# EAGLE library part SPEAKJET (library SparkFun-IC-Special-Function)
Speech synthesis chip User Manual SparkFun Products SpeakJet (COM-09578)
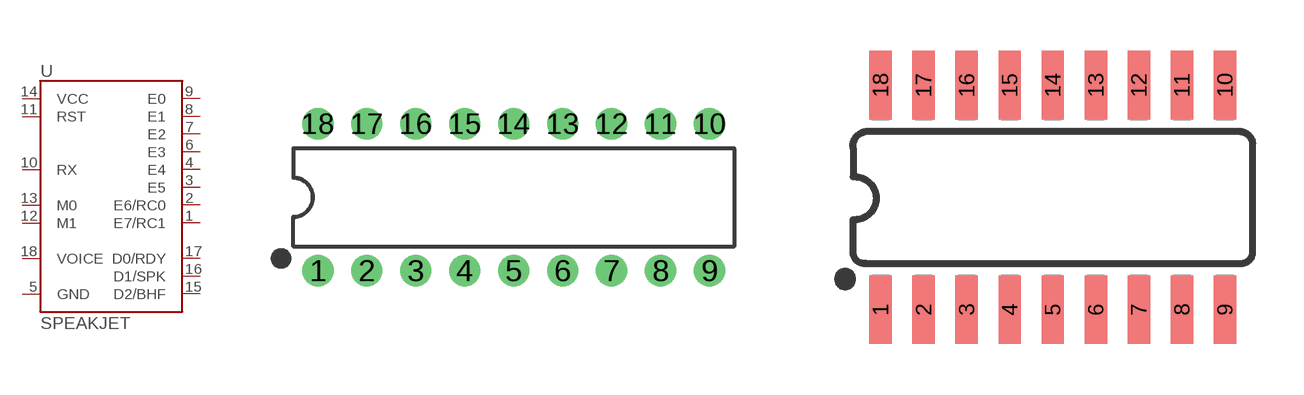
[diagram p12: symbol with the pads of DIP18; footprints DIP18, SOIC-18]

Designator prefix U

## SPEAKJETDIP (PROD_ID: IC-09512; VALUE: SPEAKJET)  [DIP18]
1  E7/RC1
2  E6/RC0
3  E5
4  E4
5  GND
6  E3
7  E2
8  E1
9  E0
10  RX
11  RST
12  M1
13  M0
14  VCC
15  D2/BHF
16  D1/SPK
17  D0/RDY
18  VOICE

## SPEAKJETSMD (PROD_ID: IC-XXXXX; VALUE: SPEAKJET)  [SOIC-18]
Pads as for DIP18

## Footprint DIP18 (pad centres in mm)
Dual In Line package type P
drill 0.813 pad 1.626: 1 -10.16,-3.81; 2 -7.62,-3.81; 3 -5.08,-3.81; 4 -2.54,-3.81; 5 0,-3.81; 6 2.54,-3.81; 7 5.08,-3.81; 8 7.62,-3.81; 9 10.16,-3.81; 10 10.16,3.81; 11 7.62,3.81; 12 5.08,3.81; 13 2.54,3.81; 14 0,3.81; 15 -2.54,3.81; 16 -5.08,3.81; 17 -7.62,3.81; 18 -10.16,3.81

## Footprint SOIC-18 (pad centres in mm)
smd 0.66 x 2.032: 1 -7.685,-3.285; 2 -6.415,-3.285; 3 -5.145,-3.285; 4 -3.875,-3.285; 5 -2.605,-3.285; 6 -1.335,-3.285; 7 -0.065,-3.285; 8 1.205,-3.285; 9 2.475,-3.285; 10 2.475,3.345; 11 1.205,3.345; 12 -0.065,3.345; 13 -1.335,3.345; 14 -2.605,3.345; 15 -3.875,3.345; 16 -5.145,3.345; 17 -6.415,3.345; 18 -7.685,3.345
